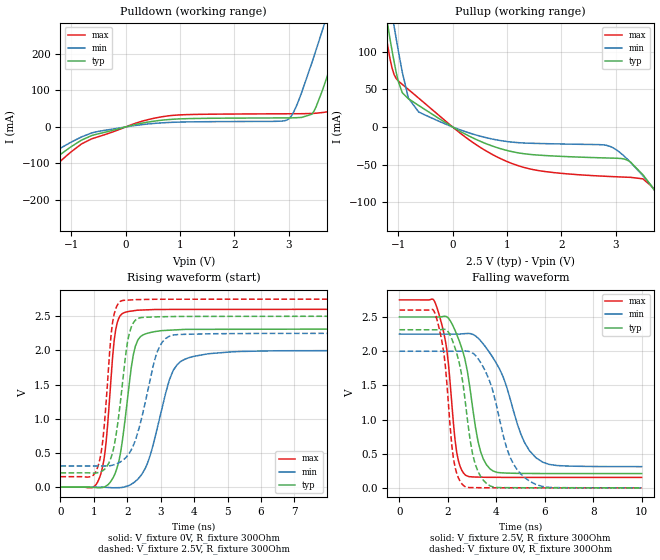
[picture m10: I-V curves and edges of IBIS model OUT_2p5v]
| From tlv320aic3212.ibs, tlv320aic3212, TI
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|   OUT_2p5v
[Model]   OUT_2p5v
Model_type   Output
Polarity   Non-Inverting
Vmeas = 1.25
Vref = 0
Cref = 5pF
Rref = 10000
|   typ   min   max
C_comp   1.397pF   1.384pF   1.430pF
[Voltage Range]   2.5   2.25   2.75
[Temperature Range]   27   125   -40
[Pullup Reference]   2.5   2.25   2.75
[Pulldown Reference]   -0   -0   -0
[Power Clamp Reference]   2.5   2.25   2.75
[GND Clamp Reference]   -0   -0   -0
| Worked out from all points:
|   slope of the pulldown table from 0 to 0.375 V, typ, clamps not added: 30.1 ohm
|   slope of the pullup table from 0 to 0.375 V, typ, clamps not added: 25.6 ohm
|   falling waveform, V_fixture 2.5V, R_fixture 300Ohm: 20-80 % time 680ps typ, 1.19ns min, 454ps max; typ from 2.5 V to 0.209 V
|   rising waveform, V_fixture 0V, R_fixture 300Ohm: 20-80 % time 371ps typ, 644ps min, 260ps max; typ from 0 V to 2.31 V
|   rising waveform, V_fixture 2.5V, R_fixture 300Ohm: 20-80 % time 352ps typ, 573ps min, 251ps max; typ from 0.209 V to 2.5 V
|   falling waveform, V_fixture 0V, R_fixture 300Ohm: 20-80 % time 591ps typ, 955ps min, 413ps max; typ from 2.31 V to 0 V
[Pulldown]
|   Voltage   I(typ)   I(min)   I(max)
-2.5V     -398.3mA   -334mA     -447.3mA
-2.125V   -228.6mA   -175mA     -272.3mA
-1.938V   -167.1mA   -129.7mA   -201.6mA
-625mV    -23.61mA   -16.48mA   -32.6mA
762.5mV   19.88mA    11.99mA    29.9mA
2.975V    24.79mA    19.61mA    36.09mA
3.425V    34.94mA    176.3mA    36.89mA
3.612V    98.03mA    262.6mA    39.36mA
3.725V    147.3mA    315.5mA    42.04mA
4.062V    305mA      476.8mA    155.2mA
4.138V    340.9mA    513mA      190mA
4.963V    742.7mA    915.3mA    589.2mA
[Pullup]
|   Voltage   I(typ)   I(min)   I(max)
-2.5V     761.5mA    811.4mA    731mA
-1.3V     182.9mA    234.3mA    151.9mA
-1.15V    116.5mA    166.2mA    89.99mA
-1.075V   86.19mA    133.3mA    69.31mA
-925mV    45.29mA    72.64mA    56.44mA
-812.5mV  37.38mA    38.17mA    49.66mA
-625mV    28.55mA    19.91mA    38.27mA
837.5mV   -27.86mA   -17.53mA   -40.47mA
2.9V      -41.28mA   -25.91mA   -65.73mA
3.5V      -63.34mA   -64.68mA   -68.86mA
4.25V     -144.1mA   -139mA     -148.8mA
4.963V    -380.8mA   -433mA     -313.2mA
[Ramp]
R_load = 300
|   typ   min   max
dV/dt_r   1.38785/3.70526e-010   1.19894/6.42227e-010   1.56086/2.60107e-010
dV/dt_f   1.37466/6.79751e-010   1.16379/1.18751e-009   1.55843/4.53966e-010
[Falling Waveform]
V_fixture = 2.5V
V_fixture_min = 2.25V
V_fixture_max = 2.75V
R_fixture = 300Ohm
C_fixture = 0F
|   Time   V(typ)   V(min)   V(max)
0s        2.5V       2.25V      2.75V
1.517ns   2.499V     2.25V      2.67V
1.954ns   2.502V     2.25V      2.026V
2.367ns   2.243V     2.249V     514.6mV
2.733ns   1.831V     2.257V     184mV
3.245ns   678.9mV    2.19V      157.4mV
3.866ns   246.4mV    1.901V     153.9mV
5.014ns   211.4mV    785.1mV    152.8mV
5.637ns   210mV      440.2mV    152.8mV
10ns      208.9mV    310.3mV    152.6mV
[Rising Waveform]
V_fixture = 0V
V_fixture_min = 0V
V_fixture_max = 0V
R_fixture = 300Ohm
C_fixture = 0F
|   Time   V(typ)   V(min)   V(max)
0s        2.105nV    249.4nV    -795.8pV
1.175ns   -9.57mV    778uV      145.5mV
1.339ns   8.685mV    -2.683mV   535.5mV
1.653ns   223.7mV    -8.484mV   2.302V
1.899ns   854.4mV    1.836mV    2.551V
2.318ns   2.155V     119.1mV    2.588V
2.691ns   2.262V     475.6mV    2.595V
3.26ns    2.295V     1.571V     2.599V
3.723ns   2.307V     1.871V     2.599V
10ns      2.313V     1.998V     2.601V
[Rising Waveform]
V_fixture = 2.5V
V_fixture_min = 2.25V
V_fixture_max = 2.75V
R_fixture = 300Ohm
C_fixture = 0F
|   Time   V(typ)   V(min)   V(max)
0s        208.9mV    310mV      152.6mV
1.112ns   211.8mV    309.4mV    289.4mV
1.28ns    245.9mV    309.3mV    743.8mV
1.562ns   511.8mV    321.7mV    2.417V
1.789ns   1.226V     367mV      2.717V
2.006ns   2.12V      461.8mV    2.736V
2.18ns    2.403V     609.8mV    2.741V
2.852ns   2.49V      1.915V     2.748V
3.26ns    2.494V     2.208V     2.748V
10ns      2.5V       2.25V      2.75V
[Falling Waveform]
|Gnd
V_fixture = 0V
V_fixture_min = 0V
V_fixture_max = 0V
R_fixture = 300Ohm
C_fixture = 0F
|   Time   V(typ)   V(min)   V(max)
0s        2.313V     1.998V     2.601V
1.471ns   2.313V     1.998V     2.549V
1.844ns   2.319V     1.998V     1.941V
2.229ns   2.116V     1.998V     429.2mV
2.642ns   1.474V     2.002V     34.63mV
3.136ns   338.1mV    1.937V     3.149mV
3.732ns   30.81mV    1.552V     1.3mV
4.573ns   2.657mV    443mV      229.3uV
5.364ns   1.174mV    99.19mV    195.9uV
10ns      2.014uV    149.2uV    -95.72nV
